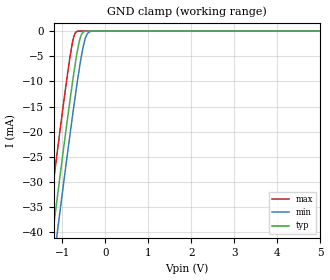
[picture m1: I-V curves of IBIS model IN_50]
| TEXAS INSTRUMENTS INCORPORATED - Standard Linear and
|   Logic Group / High Volume Linear
| EMI Filter with Integrated VCC Clamp for SIM Card Interface
| Part#   VCC Voltage Range   Package-type   #pins
|TPD5E003DPF   4.5 to 5.5V   SON   6
[IBIS Ver]   3.2
[Comment char]  |_char
[File Name]   tpd5e003.ibs
[File Rev]   1.0 | A0
[Date]   December 10, 2012
[Source]   Data created from TI-SPICE simulations at TI-SLL/HVL.
   The following is an IBIS list for the TPD3F303.
   Please contact sllibis@ti.com with questions and
   comments concerning SLL IBIS models.
[Notes]   Revision History:
   1.0: 12/10/2012
   - Initial version of the model
   - This file contains package information for the SON 6-pin
   (DPF) package as [Component] TPD5E003_DPF
   - This device can be powered at 5 volt Vcc
[Disclaimer]
| This model is designed as an aid for customers of Texas Instruments.
| TI and its licensors and suppliers make no warranties, either expressed
| or implied, with respect to this  model, including the warranties of
| merchantability or fitness for a particular purpose. The model is
| provided solely on an "as is" basis. The entire risk as to its quality
| and performance is with the customer.
[Copyright]
| (C) Copyright 2011 Texas Instruments Incorporated. All rights reserved.
| Component TPD5E003_DPF 6-PIN SON
[Component]   TPD5E003_DPF
[Manufacturer]   Texas Instruments, Inc.
[Package]
|   typ   min   max
R_pkg   6.141e-02   1.500e-02   7.441e-02
L_pkg   5.439e-10   6.250e-12   6.642e-10
C_pkg   1.493e-13   8.600e-14   3.412e-13
[Pin]   signal_name   model_name   R_pin   L_pin   C_pin
1   IO1   IN_50   7.220e-02   6.416e-10   1.173e-13
2   GND   POWER   1.500e-03   6.250e-12   8.600e-14
3   IO2   IN_50   7.441e-02   6.642e-10   1.183e-13
4   IO3   IN_50   7.424e-02   6.568e-10   1.190e-13
5   IO4   IN_50   7.292e-02   6.422e-10   1.141e-13
6   IO5   IN_50   7.310e-02   6.524e-10   3.412e-13
| Models and submodels in the file (1): IN_50 (Input)
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[Model]   IN_50
Model_type  Input
Vinl=1.75
Vinh=3.25
| variable   typ   min   max
C_comp   10pF   8pF   12pF
[Temperature Range]   40   100   -40
| Ambient temperature   25   85   -40
[Voltage range]   5   4.5   5.5
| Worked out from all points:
|   GND clamp passes 1 mA (typ) near -0.57 V on its own axis
[GND Clamp]
| IN_50
|   Voltage   I(typ)   I(min)   I(max)
-5V       -304.8mA   -311.4mA   -296.4mA
-1.35V    -48.74mA   -55.7mA    -39.68mA
-1.23V    -40.56mA   -47.53mA   -31.47mA
-1.13V    -33.79mA   -40.77mA   -24.71mA
-1.095V   -31.44mA   -38.42mA   -22.36mA
-800mV    -12.27mA   -19.04mA   -3.895mA
-730mV    -8.099mA   -14.67mA   -974.8uA
-665mV    -4.585mA   -10.76mA   -86.23uA
-580mV    -1.209mA   -6.047mA   -1.421uA
-495mV    -110.6uA   -2.294mA   -21.2nA
-350mV    -579.4nA   -83.81uA   -365.9pA
5V        5.011nA    6.712nA    5.01nA
